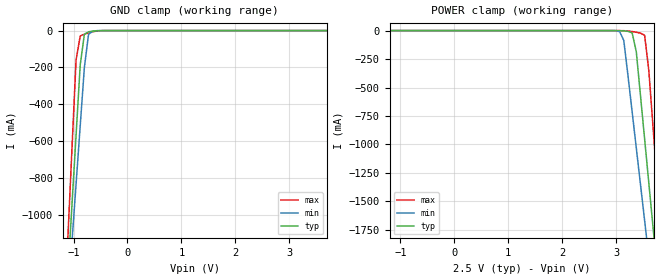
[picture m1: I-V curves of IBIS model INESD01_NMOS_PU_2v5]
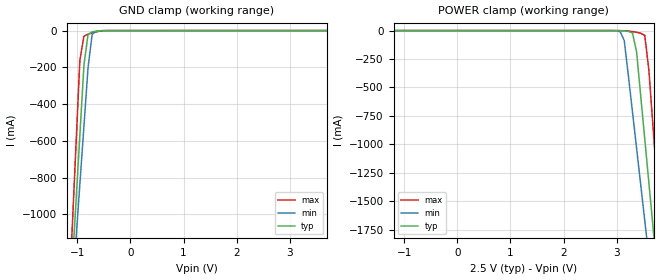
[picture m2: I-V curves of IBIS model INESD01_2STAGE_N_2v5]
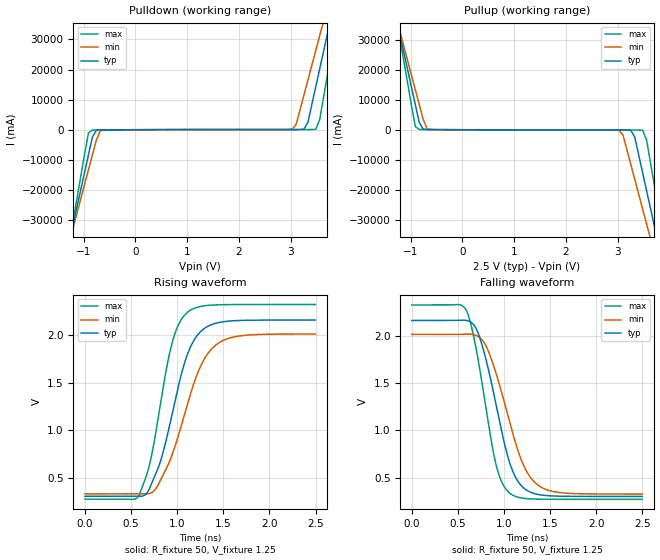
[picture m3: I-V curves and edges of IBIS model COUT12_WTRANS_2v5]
|   This file is an IBIS representation of the   |
|   Integrated Device Technology,Inc.   |
|   ICS840051I   |
|   FEMTOCLOCKS CRYSTAL-TOLVCMOS/LVTTL CLOCK GENERATOR   |
[IBIS Ver]   4.1
[File name]   840051i.ibs
[File Rev]   1.0
[Date]   15 Jun 2009 | Last modified
|   May 17 2006 | Generated
[Source]   Originated at Integrated Devices Technology, Inc.
[Disclaimer]
IDT hereby grants the user of this IBIS model a non-exclusive,
nontransferable license to use this IBIS model under the following terms.
Before using this IBIS model, the user should read this license.
If the user does not accept these terms,  the IBIS model should be
returned to IDT within 30 days.
   The user is granted this license only to use the IBIS model and
is not granted rights to sell, load, rent, lease or license the IBIS
model in whole or in part, or in modified form to anyone other than
user. User may modify the IBIS model to suit its specific
applications but rights to derivative works and such modifications
shall belong to IDT.
   This IBIS model is provided on an "AS IS" basis and IDT makes
absolutely no warranty with respect to the information contained
herein. IDT DISCLAIMS AND CUSTOMER WAIVES ALL WARRANTIES, EXPRESS
OR IMPLIED, INCLUDING WARRANTIES OF MERCHANTABILITY OR FITNESS FOR
A PARTICULAR PURPOSE. The entire risk as to quality and performance
is with the Customer. ACCORDINGLY, IN NO EVENT SHALL THE COMPANY BE
LIABLE FOR ANY DAMAGES, WHETHER IN CONTRACT OR TORT,INCLUDING ANY
LOST PROFITS OR OTHER INCIDENTAL, CONSEQUENTIAL, EXEMPLARY, OR
PUNITIVE DAMAGES ARISING OUT OF THE USE OR APPLICATION OF THE IBIS
model provided in this package. Further, IDT reserves the right to
make changes without notice to any product herein to improve
reliability, function, or design. IDT does not convey any license
under patent rights or any other intellectual property rights,
including those of third parties.
   IDT is not obligated to provide maintenance or support
for the licensed IBIS model.
[Copyright]   Copyright 2007 by Integrated Device Technology,Inc
[Component]   ICS840051GI
[Manufacturer] Integrated Devices Technology, Inc.
[Package]
|TSSOP 8 Lead
|   typ   min   max
R_pkg   52.5m   48.8m   56.2m
L_pkg   1.381nH   1.275nH   1.486nH
C_pkg   0.236pF   0.230pF   0.242pF
[Pin] signal_name  model_name   R_pin   L_pin   C_pin
1   VDDA   POWER   56.2m   1.486n   0.242p
2   OE   INESD01_NMOS_PU   48.8m   1.275n   0.230p
3   XTAL_OUT   NC   48.8m   1.275n   0.230p
4   XTAL_IN   NC   56.2m   1.468n   0.242p
5   FRE_SEL   INESD01_2STAGE_N   56.2m   1.486n   0.242p
6   GND   GND   48.8m   1.275n   0.230p
7   Q0   COUT12_WTRANS   48.8m   1.275n   0.230p
8   VDD   POWER   56.2m   1.468n   0.242p
[Model Selector] INESD01_NMOS_PU
INESD01_NMOS_PU_2v5  Buffer selection for 2v5
INESD01_NMOS_PU_3v3  Buffer selection for 3v3
[Model Selector] INESD01_2STAGE_N
INESD01_2STAGE_N_2v5  Buffer selection for 2v5
INESD01_2STAGE_N_3v3  Buffer selection for 3v3
[Model Selector] COUT12_WTRANS
COUT12_WTRANS_2v5  Buffer selection for 2v5
COUT12_WTRANS_3v3  Buffer selection for 3v3
| Models and submodels in the file (6): INESD01_NMOS_PU_2v5 (Input), INESD01_2STAGE_N_2v5 (Input), COUT12_WTRANS_2v5 (Output), INESD01_NMOS_PU_3v3 (Input), INESD01_2STAGE_N_3v3 (Input), COUT12_WTRANS_3v3 (Output)
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[Model] INESD01_NMOS_PU_2v5
Model_type   Input
Polarity   Non-Inverting
Vinl = 0.5V
Vinh = 1.1V
|   typ   min   max
C_comp   2pF   1.5pF   2.5pF
|   typ   min   max
[Voltage range]  2.5V   2.375V   2.625V
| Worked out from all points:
|   GND clamp passes 1 mA (typ) near -0.57 V on its own axis
[GND_clamp]
|Voltage I(typ)   I(min)   I(max)
-2.5V     -8.263A    -7.237A    -9.981A
-1.108V   -1.337A    -1.473A    -1.142A
-1.031V   -953.1mA   -1.154A    -651.2mA
-953.6mV  -569.5mA   -835mA     -160.3mA
-876.3mV  -186.2mA   -516.8mA   -29.47mA
-799mV    -19.59mA   -199.2mA   -19.31mA
-721.6mV  -6.713mA   -20.65mA   -12.35mA
-644.3mV  -2.945mA   -2.694mA   -6.489mA
-489.7mV  -219.7uA   -96.65uA   -544uA
5V        555.4pA    974.3pA    139.3pA
[POWER_clamp]
|Voltage   I(typ)   I(min)   I(max)
-2.5V     555.4pA    852.5pA    162.9pA
3.067V    -971.3uA   -8.981mA   -175.9uA
3.144V    -2.945mA   -87.2mA    -1.018mA
3.299V    -19.59mA   -713mA     -8.571mA
3.376V    -186.2mA   -1.031A    -14.91mA
3.454V    -569.5mA   -1.35A     -22.33mA
3.531V    -953.1mA   -1.669A    -41.51mA
3.608V    -1.337A    -1.989A    -348.5mA
3.686V    -1.721A    -2.309A    -839.4mA
3.763V    -2.106A    -2.628A    -1.33A
3.84V     -2.49A     -2.948A    -1.822A
5V        -8.263A    -7.755A    -9.188A
[Model] INESD01_2STAGE_N_2v5
Model_type   Input
Polarity   Non-Inverting
Vinl = .8V
Vinh = 2V
|   typ   min   max
C_comp   2pF   1.5pF   2.5pF
|   typ   min   max
[Voltage range]  2.5V   2.375V   2.625V
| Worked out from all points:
|   GND clamp passes 1 mA (typ) near -0.56 V on its own axis
[GND_clamp]
|Voltage   I(typ)   I(min)   I(max)
-2.5V     -8.269A    -7.245A    -9.986A
-1.108V   -1.338A    -1.475A    -1.143A
-1.031V   -954.2mA   -1.155A    -652.3mA
-953.6mV  -570.3mA   -836.3mA   -161.2mA
-876.3mV  -186.9mA   -517.7mA   -30.19mA
-799mV    -20.06mA   -199.8mA   -19.86mA
-721.6mV  -7.024mA   -20.98mA   -12.73mA
-644.3mV  -3.118mA   -2.836mA   -6.727mA
-489.7mV  -245.9uA   -116.3uA   -585.7uA
5V        96.94uA    121.2uA    75.12uA
[POWER_clamp]
|Voltage   I(typ)   I(min)   I(max)
-2.5V     96.94uA    118.2uA    76.99uA
3.067V    -1.047mA   -9.228mA   -195uA
3.144V    -3.118mA   -87.68mA   -1.083mA
3.299V    -20.06mA   -714.1mA   -8.863mA
3.376V    -186.9mA   -1.033A    -15.35mA
3.454V    -570.3mA   -1.352A    -22.94mA
3.531V    -954.2mA   -1.672A    -42.29mA
3.608V    -1.338A    -1.991A    -349.4mA
3.686V    -1.723A    -2.311A    -840.5mA
3.763V    -2.108A    -2.632A    -1.332A
3.84V     -2.492A    -2.952A    -1.823A
5V        -8.269A    -7.765A    -9.192A
[Model] COUT12_WTRANS_2v5
Model_type   Output
Polarity   Non-Inverting
|   typ   min   max
C_comp   2pF   1.5pF   2.5pF
Vmeas = 1.25V
Rref = 50
Cref = 50
Vref = 1.25V
|   typ   min   max
[Voltage range]   2.5V   2.375V   2.625V
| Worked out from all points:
|   slope of the pulldown table from 0 to 0.375 V, typ, clamps not added: 16.5 ohm
|   slope of the pullup table from 0 to 0.375 V, typ, clamps not added: 18.9 ohm
|   rising waveform, R_fixture 50, V_fixture 1.25: 20-80 % time 288ps typ, 340ps min, 232ps max; typ from 0.303 V to 2.16 V
|   falling waveform, R_fixture 50, V_fixture 1.25: 20-80 % time 262ps typ, 307ps min, 215ps max; typ from 2.16 V to 0.303 V
[Pulldown]
|Voltage   I (typ)   I (min)   I (max)
-2.5V     -132.4A    -116.6A    -159.3A
-1.288V   -37.91A    -37.91A    -38.44A
-1.212V   -32A       -32.99A    -30.89A
-909.1mV  -8.368A    -13.32A    -1.073A
-833.3mV  -2.461A    -8.397A    -92.21mA
-606.1mV  -40.23mA   -65.84mA   -45.64mA
3.03V     52.18mA    193.7mA    61.66mA
3.333V    2.453A     16.49A     62.14mA
3.485V    14.25A     26.32A     148.7mA
3.712V    31.96A     41.06A     18.39A
3.864V    43.76A     50.89A     33.49A
5V        132.3A     124.6A     146.7A
[Pullup]
|Voltage   I (typ)   I (min)   I (max)
-2.5V     132.4A     116.6A     159.3A
-1.288V   37.88A     37.89A     38.42A
-1.212V   31.98A     32.97A     30.87A
-909.1mV  8.357A     13.31A     1.064A
-833.3mV  2.454A     8.39A      87.48mA
-606.1mV  38.86mA    63.99mA    46.61mA
3.03V     -57.97mA   -201.8mA   -71.64mA
3.333V    -2.473A    -16.52A    -77.44mA
3.485V    -14.28A    -26.35A    -176.1mA
3.712V    -32A       -41.11A    -18.44A
3.864V    -43.82A    -50.94A    -33.55A
5V        -132.4A    -124.7A    -146.8A
[Ramp]
|   typ   min   max
dV/dt_r   1.486/0.453n   1.348/0.531n   1.642/0.366n
dV/dt_f   1.489/0.396n   1.35/0.466n   1.645/0.325n
R_load =   50.0000
[Rising Waveform]
R_fixture = 50
V_fixture = 1.25   |Vcc_typ
V_fixture_min = 1.1875 |Vcc_min
V_fixture_max = 1.3125 |Vcc_max
C_fixture = 0.0p
| Time   typ   min   max
0s        302.6mV    327.8mV    272.2mV
583.1ps   301.6mV    328mV      307.8mV
700.7ps   387.7mV    332.6mV    637.8mV
805.8ps   632.8mV    446.5mV    1.199V
951ps     1.196V     756mV      1.941V
1.021ns   1.496V     968.5mV    2.126V
1.109ns   1.791V     1.264V     2.239V
1.279ns   2.06V      1.723V     2.308V
1.474ns   2.139V     1.933V     2.322V
2.498ns   2.16V      2.013V     2.324V
[Falling Waveform]
R_fixture = 50
V_fixture = 1.25   |Vcc_typ
V_fixture_min = 1.1875 |Vcc_min
V_fixture_max = 1.3125 |Vcc_max
C_fixture = 0.0p
| Time   typ   min   max
0s        2.16V      2.013V     2.324V
590.6ps   2.162V     2.016V     2.267V
653.2ps   2.133V     2.014V     2.069V
728.2ps   2.003V     1.986V     1.696V
908.4ps   1.296V     1.617V     657.8mV
976ps     982.4mV    1.393V     452.7mV
1.059ns   665.1mV    1.096V     339.6mV
1.224ns   383.1mV    606mV      281.8mV
1.406ns   317.5mV    397.7mV    273.6mV
2.498ns   302.6mV    327.8mV    272.2mV
